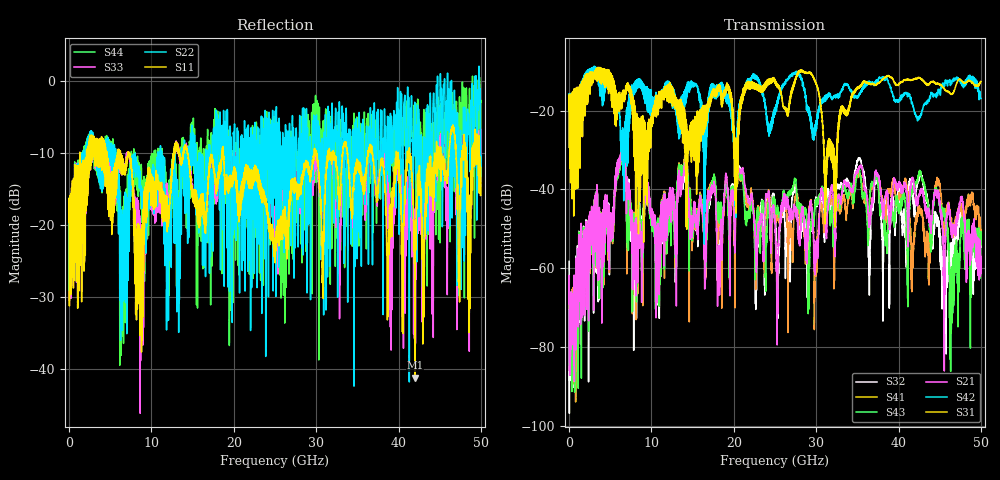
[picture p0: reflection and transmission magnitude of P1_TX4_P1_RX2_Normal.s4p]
!Keysight Technologies,N5225B,MY57041031,A.13.20.10
!Date: Friday, May 31, 2019 11:15:43
!Correction: S11(Full 4 Port(1,2,3,4))
!S12(Full 4 Port(1,2,3,4))
!S13(Full 4 Port(1,2,3,4))
!S14(Full 4 Port(1,2,3,4))
!S21(Full 4 Port(1,2,3,4))
!S22(Full 4 Port(1,2,3,4))
!S23(Full 4 Port(1,2,3,4))
!S24(Full 4 Port(1,2,3,4))
!S31(Full 4 Port(1,2,3,4))
!S32(Full 4 Port(1,2,3,4))
!S33(Full 4 Port(1,2,3,4))
!S34(Full 4 Port(1,2,3,4))
!S41(Full 4 Port(1,2,3,4))
!S42(Full 4 Port(1,2,3,4))
!S43(Full 4 Port(1,2,3,4))
!S44(Full 4 Port(1,2,3,4))
!S4P File: Measurements: <S11,S12,S13,S14>,
!<S21,S22,S23,S24>,
!<S31,S32,S33,S34>,
!<S41,S42,S43,S44>:
# Hz S  dB  R 50.0
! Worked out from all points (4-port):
!   5000 points, 10 MHz to 50 GHz, reference 50 ohm
!   strongest paths, dB at 10 MHz, 12.51 GHz, 25.01 GHz, 37.51 GHz, 50 GHz:
!     S31: -19.7, -17.6, -12.9, -13.1, -12.6
!     S42: -19.4, -16.3, -19.3, -12.4, -16.9
!     S21: -69.1, -41.3, -49.2, -36.9, -59.0
!     S43: -65.6, -42.7, -43.6, -38.5, -52.6
!     S41: -71.4, -42.3, -45.3, -37.2, -50.2
!     S32: -58.3, -41.6, -44.9, -38.4, -51.2
!   lowest |S11| = -41.1 dB at 42 GHz (marker M1), VSWR 1.02, Z = 49.3 + j0.499 ohm
!   |S11| at or under -10 dB: 7.336 GHz to 12.7 GHz (5.362 GHz wide, 53.5 % of centre); 14.41 GHz to 18.57 GHz (4.157 GHz wide, 25.2 % of centre); 18.74 GHz to 29.76 GHz (11.02 GHz wide, 45.4 % of centre)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
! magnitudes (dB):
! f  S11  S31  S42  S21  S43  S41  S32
! 10 MHz  -19.5  -19.7  -19.4  -69.1  -65.6  -71.4  -58.3
! 6.53 GHz  -11.0  -15.9  -32.6  -28.4  -29.1  -28.8  -28.4
! 10.78 GHz  -14.1  -18.6  -18.7  -65.9  -56.8  -56.1  -64.9
! 29.22 GHz  -12.6  -10.3  -21.6  -44.8  -56.0  -44.1  -51.2
! 32.24 GHz  -10.4  -35.8  -16.5  -50.5  -46.9  -57.6  -49.4
! 42 GHz  -41.1  -11.9  -20.5  -40.6  -39.1  -49.6  -45.1
! 50 GHz  -12.0  -12.6  -16.9  -59.0  -52.6  -50.2  -51.2
